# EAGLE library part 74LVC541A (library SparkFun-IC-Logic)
74LVC541A IC OCTAL BUFFER, SCHMITT TRIGGER The 74LVC541A is an 8-bit buffer/line driver with 3-state outputs. The device features two output enables (OE1 and OE2). A HIGH on OEn causes the associated outputs to assume a high-impedance OFF-state . Inputs can be driven from either 3.3 V or 5 V devices. This feature allows the use of these devices as translators in mixed 3.3 V and 5 V environments. SparkFun Products: MicroMod Function u-blox ZED-F9P board
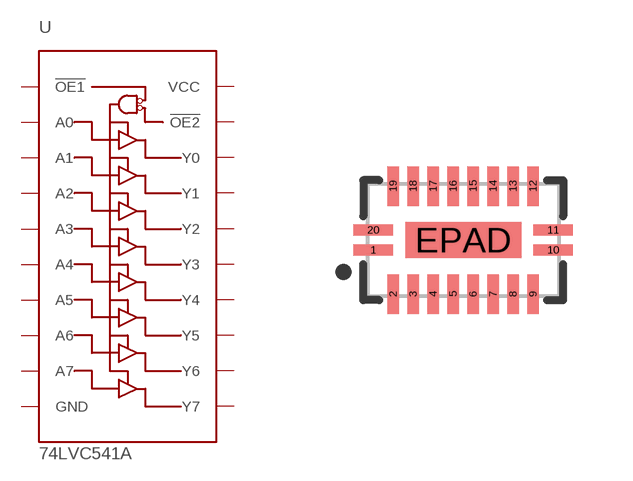
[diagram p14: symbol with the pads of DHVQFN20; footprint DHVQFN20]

Designator prefix U

## 74LVC541ABQ (PROD_ID: IC-16698; VALUE: 74LVC541A)  [DHVQFN20]
1  !OE1!  in
2  A0  in
3  A1  in
4  A2  in
5  A3  in
6  A4  in
7  A5  in
8  A6  in
9  A7  in
10  GND  pwr
11  Y7  out
12  Y6  out
13  Y5  out
14  Y4  out
15  Y3  out
16  Y2  out
17  Y1  out
18  Y0  out
19  !OE2!  in
20  VCC  pwr
EPAD  GND  pwr

## Footprint DHVQFN20 (pad centres in mm)
DHVQFN20 - 20-pin plastic, leadless, very thin quad flat package Mechanical Specifications: Pad Size: 0.29mm x 0.9mm Pin count: 20 Pin pitch: 0.5mm Package Size: 2.5mm x 4.5mm Datasheet referenced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
smd 0.99 x 0.28: 1 -2.25,-0.25; 10 2.25,-0.25; 11 2.25,0.25; 20 -2.25,0.25
smd 0.28 x 0.99: 2 -1.75,-1.35; 3 -1.25,-1.35; 4 -0.75,-1.35; 5 -0.25,-1.35; 6 0.25,-1.35; 7 0.75,-1.35; 8 1.25,-1.35; 9 1.75,-1.35; 12 1.75,1.35; 13 1.25,1.35; 14 0.75,1.35; 15 0.25,1.35; 16 -0.25,1.35; 17 -0.75,1.35; 18 -1.25,1.35; 19 -1.75,1.35
smd 2.9 x 0.9: EPAD 0,0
